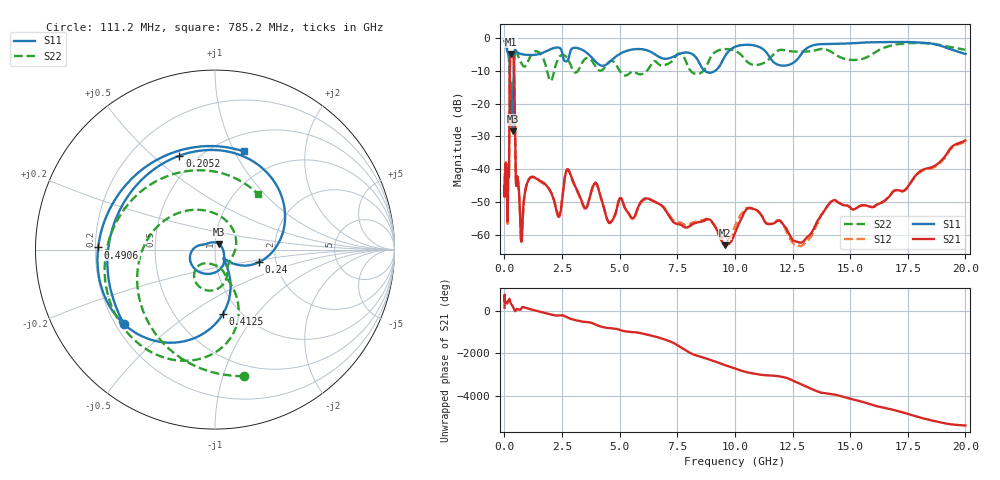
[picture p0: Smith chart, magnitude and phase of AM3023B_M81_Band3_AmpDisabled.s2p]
!Agilent Technologies,E8364B,MY43040894,A.07.50.67
!Agilent E8364B: A.07.50.67
!Date: Tuesday, October 27, 2020 10:39:11
!Correction: S11(Full 2 Port(1,2))
!S21(Full 2 Port(1,2))
!S12(Full 2 Port(1,2))
!S22(Full 2 Port(1,2))
!S2P File: Measurements: S11, S21, S12, S22:Log Frequency Sweep
# Hz S  dB  R 50
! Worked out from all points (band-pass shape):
!   3201 points, 10 MHz to 20 GHz, reference 50 ohm
!   highest |S21| = -4.79 dB at 283.4 MHz (marker M1); lowest = -63.3 dB at 9.577 GHz (marker M2)
!   |S21| within 3 dB of the highest: 241.7 MHz to 412.3 MHz (170.6 MHz wide, 52.2 % of centre)
!   lowest |S11| = -28.4 dB at 361.1 MHz (marker M3), VSWR 1.08, Z = 52 + j3.3 ohm
!   |S11| at or under -10 dB: 237.2 MHz to 408.8 MHz (171.6 MHz wide, 53.1 % of centre); 8.711 GHz to 9.128 GHz (416.5 MHz wide, 4.67 % of centre)
!   |S22| runs from -21.6 to -0.9 dB; largest |S21 - S12| = 0.01
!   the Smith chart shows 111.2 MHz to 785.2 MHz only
!   S11 on the Smith chart (normalised r, x): 111.2 MHz: 0.23, -0.34; 205.2 MHz: 0.40, +0.61; 240 MHz: 1.63, -0.24; 412.5 MHz: 0.84, -0.69; 490.6 MHz: 0.21, +0.01; 785.2 MHz: 0.67, +1.09
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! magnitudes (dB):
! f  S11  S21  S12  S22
! 10 MHz  -0.7  -45.2  -46.3  -0.9
! 35.55 MHz  -1.3  -40.6  -40.4  -1.2
! 111.2 MHz  -3.7  -42.3  -42.7  -2.8
! 126.1 MHz  -4.0  -47.9  -47.4  -3.2
! 141.3 MHz  -4.3  -55.8  -56.7  -3.7
! 205.2 MHz  -5.0  -38.4  -38.2  -7.4
! 240 MHz  -11.8  -8.4  -8.4  -17.3
! 283.4 MHz  -18.5  -4.8  -4.8  -13.7
! 361.1 MHz  -28.4  -5.0  -5.0  -20.7
! 412.5 MHz  -8.9  -7.8  -7.9  -10.1
! 447.2 MHz  -3.7  -19.2  -19.2  -3.9
! 490.6 MHz  -3.7  -41.0  -40.9  -3.6
! 785.2 MHz  -4.9  -56.6  -57.0  -8.2
! 1.015 GHz  -5.1  -43.7  -43.8  -7.2
! 1.59 GHz  -4.6  -43.7  -43.9  -4.9
! 2.358 GHz  -2.8  -54.5  -54.0  -6.0
! 2.765 GHz  -6.5  -40.1  -40.2  -6.5
! 5.639 GHz  -3.3  -54.6  -54.8  -10.2
! 9.577 GHz  -5.3  -63.3  -61.6  -3.3
! 10.73 GHz  -2.0  -52.0  -52.1  -8.0
! 12.92 GHz  -4.4  -62.3  -63.4  -4.0
! 20 GHz  -4.8  -31.2  -31.5  -3.5
